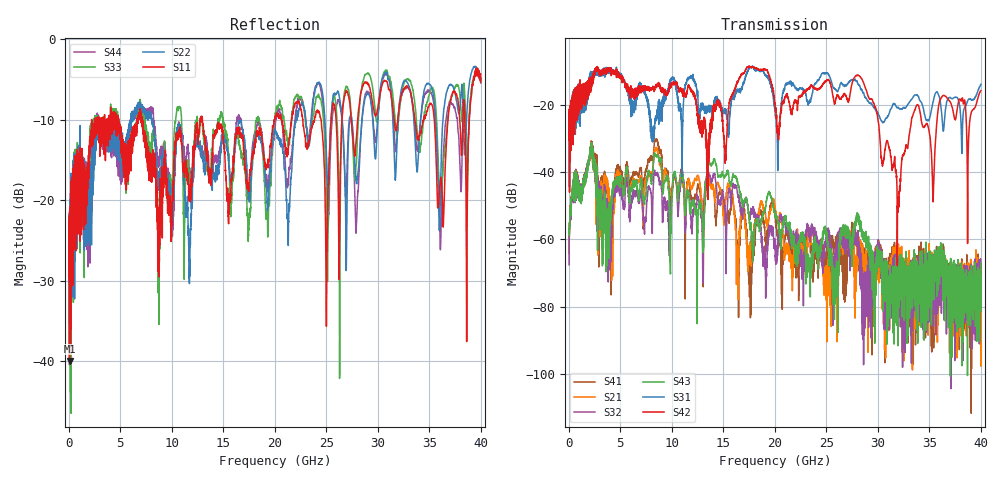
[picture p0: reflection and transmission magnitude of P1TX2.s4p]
!Agilent Technologies,N5245A,MY49151084,A.09.20.08
!Agilent N5245A: A.09.20.08
!Date: Thursday, March 01, 2012 14:35:31
!Correction: S11(Full 4 Port(1,2,3,4))
!S12(Full 4 Port(1,2,3,4))
!S13(Full 4 Port(1,2,3,4))
!S14(Full 4 Port(1,2,3,4))
!S21(Full 4 Port(1,2,3,4))
!S22(Full 4 Port(1,2,3,4))
!S23(Full 4 Port(1,2,3,4))
!S24(Full 4 Port(1,2,3,4))
!S31(Full 4 Port(1,2,3,4))
!S32(Full 4 Port(1,2,3,4))
!S33(Full 4 Port(1,2,3,4))
!S34(Full 4 Port(1,2,3,4))
!S41(Full 4 Port(1,2,3,4))
!S42(Full 4 Port(1,2,3,4))
!S43(Full 4 Port(1,2,3,4))
!S44(Full 4 Port(1,2,3,4))
!S4P File: Measurements: <S11,S12,S13,S14>,
!<S21,S22,S23,S24>,
!<S31,S32,S33,S34>,
!<S41,S42,S43,S44>:
# Hz S  dB  R 50
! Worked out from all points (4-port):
!   3996 points, 50 MHz to 40 GHz, reference 50 ohm
!   strongest paths, dB at 50 MHz, 10.04 GHz, 20.03 GHz, 30.02 GHz, 40 GHz:
!     S42: -25.3, -13.5, -19.4, -24.4, -15.7
!     S31: -25.4, -12.1, -21.9, -22.2, -13.8
!     S43: -56.7, -46.0, -53.5, -64.2, -67.1
!     S32: -67.6, -45.1, -61.9, -61.6, -74.4
!     S21: -63.5, -44.8, -50.1, -66.2, -68.6
!     S41: -64.2, -45.8, -52.6, -61.7, -70.1
!   lowest |S11| = -40.0 dB at 90 MHz (marker M1), VSWR 1.02, Z = 50.7 + j0.749 ohm
!   |S11| at or under -10 dB: start of sweep to 2.239 GHz; 7.17 GHz to 12.77 GHz (5.596 GHz wide, 56.1 % of centre); 12.98 GHz to 19.93 GHz (6.945 GHz wide, 42.2 % of centre)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
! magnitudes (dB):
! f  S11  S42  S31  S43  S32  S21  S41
! 50 MHz  -24.1  -25.3  -25.4  -56.7  -67.6  -63.5  -64.2
! 90 MHz  -40.0  -46.0  -44.4  -55.3  -57.0  -56.0  -54.9
! 8.49 GHz  -19.0  -14.4  -23.5  -35.1  -40.3  -32.8  -30.2
! 17.59 GHz  -16.6  -8.6  -8.8  -56.9  -54.1  -66.9  -74.5
! 28.08 GHz  -9.4  -11.1  -13.9  -54.3  -64.8  -63.0  -62.8
! 32.03 GHz  -9.0  -48.1  -20.9  -69.5  -73.8  -65.5  -77.3
! 40 GHz  -5.3  -15.7  -13.8  -67.1  -74.4  -68.6  -70.1
